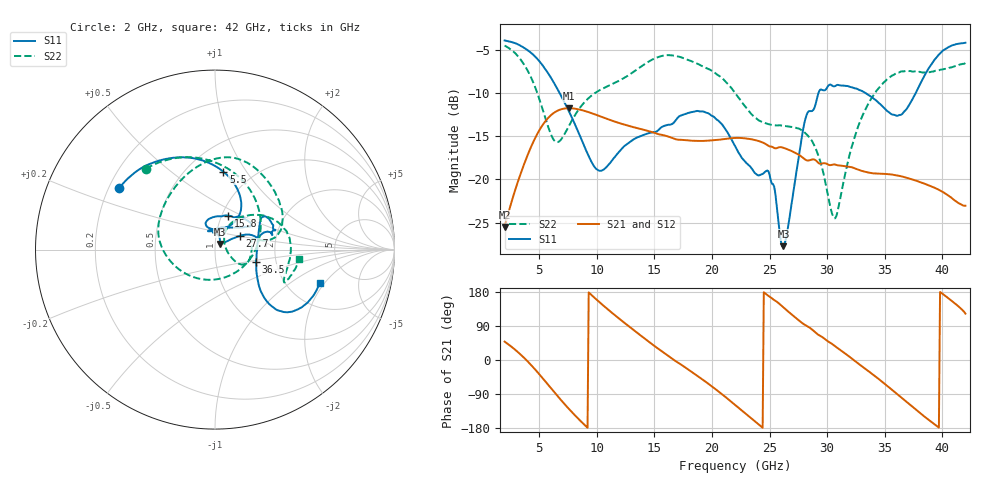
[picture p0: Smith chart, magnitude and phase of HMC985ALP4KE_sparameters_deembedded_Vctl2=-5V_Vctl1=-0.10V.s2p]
!s2p File: Measurements: S11, S21, S12, S22
# GHz S dB R 50.0
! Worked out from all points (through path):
!   401 points, 2 GHz to 42 GHz, reference 50 ohm
!   highest |S21| = -11.77 dB at 7.6 GHz (marker M1); lowest = -25.5 dB at 2 GHz (marker M2)
!   lowest |S11| = -27.7 dB at 26.2 GHz (marker M3), VSWR 1.09, Z = 52.6 + j3.37 ohm
!   |S11| at or under -10 dB: 6.767 GHz to 29.25 GHz (22.49 GHz wide, 125 % of centre); 33.3 GHz to 37.7 GHz (4.395 GHz wide, 12.4 % of centre)
!   |S22| runs from -24.5 to -4.5 dB; largest |S21 - S12| = 0.00023
!   S11 on the Smith chart (normalised r, x): 2 GHz: 0.24, +0.28; 5.5 GHz: 0.74, +0.79; 15.8 GHz: 1.07, +0.42; 27.7 GHz: 1.30, +0.21; 36.5 GHz: 1.57, -0.23; 42 GHz: 3.02, -1.81
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2  -3.95 147.1  -25.50 48.5  -25.51 48.5  -4.54 130.5
3.6  -4.73 120.4  -18.57 8.3  -18.57 8.3  -6.56 85.0
5.5  -7.20 83.9  -13.34 -55.2  -13.35 -55.2  -12.75 2.4
6.5  -9.35 66.7  -12.12 -91.7  -12.13 -91.7  -15.68 -69.4
7.6  -12.18 55.4  -11.77 -129.7  -11.78 -129.7  -13.78 -136.1
8.7  -15.48 56.4  -11.99 -164.2  -12.00 -164.2  -11.44 -170.4
10.2  -18.98 85.5  -12.66 153.5  -12.66 153.5  -9.73 165.1
11.9  -16.87 110.2  -13.47 110.2  -13.47 110.2  -8.63 141.7
15.4  -14.24 76.1  -14.79 28.4  -14.80 28.4  -5.83 87.5
15.8  -13.84 69.2  -14.89 19.5  -14.90 19.5  -5.70 82.5
19.4  -12.24 33.9  -15.54 -56.3  -15.54 -56.3  -7.06 35.7
22  -16.12 51.7  -15.21 -118.3  -15.21 -118.2  -9.99 10.3
24.9  -19.05 104.2  -16.11 169.2  -16.12 169.2  -13.61 13.3
26.2  -27.70 50.9  -16.34 138.7  -16.35 138.8  -13.81 -1.4
27.7  -15.98 29.0  -17.29 100.7  -17.30 100.7  -14.25 -21.6
28.7  -12.09 13.0  -17.70 80.1  -17.70 80.2  -15.59 -29.7
30.7  -9.22 21.0  -18.28 36.0  -18.29 36.0  -24.48 22.2
32.9  -9.72 34.2  -18.97 -13.9  -18.98 -13.9  -13.16 52.9
35.4  -12.27 11.5  -19.40 -73.0  -19.41 -72.9  -8.24 22.1
36.5  -12.46 -16.5  -19.66 -100.7  -19.67 -100.7  -7.52 8.1
39.5  -5.91 -42.8  -21.07 -173.8  -21.07 -173.8  -7.44 -24.9
42  -4.21 -17.6  -23.03 122.4  -23.04 122.3  -6.54 -6.2
